PROGRAM MAIN
VAR
	fbSocketConnect   	: FB_SocketConnect;(*TCP/IP建立连接的功能块*)
	fbSocketSend      	: FB_SocketSend;(*TCP/IP的发送功能块*)
	fbSocketReceive   	: FB_SocketReceive;(*TCP/IP的写入的功能块*)
	fbSocketClose     	: FB_SocketClose;(*TCP/IP的关闭建立连接的功能块*)
    bExecute          	: BOOL;(*TCP/IP建立连接的执行位*)
    hSocket           	: T_HSOCKET;(*TCP/IP的句柄*)
	arrSendData			: ARRAY[1..4] OF WORD := [16#1111, 16#2222, 16#3333, 16#4444];(*TCP/IP发送数组*)
	bSend				: BOOL;(*TCP/IP发送的执行位*)
	bRecieve          	: BOOL;(*TCP/IP接收的执行位*)
	arrRecieveData    	: ARRAY[1..4] OF WORD;(*TCP/IP接收数组*)
	bClose            	: BOOL;(*TCP/IP关闭连接的执行位*)
END_VAR

/////////////////////////////////////////////////////////
//注意：/////////////////////////////////////////////////
//该例程序仅供初学者入门学习使用/////////////////////////
//差错在所难免，无法保证绝对正确并完全满足您的使用需求///
//欢迎您提出改进建议。联系邮箱：Support@Beckhoff.com.cn//
/////////////////////////////////////////////////////////

fbSocketConnect(
	sSrvNetId:= , 
	sRemoteHost:='169.254.0.1', //TCP/IP Server的IP地址169.254.0.1
	nRemotePort:=6000 , 		//TCP/IP Server的I端口号6000
	bExecute:= bExecute, 		//TCP/IP连接的执行位*)
	tTimeout:=T#1S , 
	bBusy=> , 
	bError=> , 
	nErrId=> , 
	hSocket=>hSocket );			//通过SocketConnect获取句柄，供后续FB使用
	
fbSocketSend(
	sSrvNetId:= , 
	hSocket:=hSocket , 			//TCP/IP的句柄
	cbLen:=SIZEOF(arrSendData) ,//TCP/IP发送数据的长度
	pSrc:=ADR (arrSendData), 	//TCP/IP发送数据的指针起始地址
	bExecute:=bSend, 			//TCP/IP发送的执行位
	tTimeout:= T#1S, 
	bBusy=> , 
	bError=> , 
	nErrId=> );
	
fbSocketReceive(
	sSrvNetId:= , 
	hSocket:=hSocket , 				//TCP/IP的句柄
	cbLen:=SIZEOF(arrRecieveData) , //TCP/IP接收数据的长度
	pDest:=ADR (arrRecieveData) , 	//TCP/IP接收数据的指针起始地址
	bExecute:=bRecieve, 			//TCP/IP接收的执行位
	tTimeout:= T#1S , 
	bBusy=> , 
	bError=> , 
	nErrId=> , 
	nRecBytes=> );
	
fbSocketClose(
	sSrvNetId:= , 
	hSocket:=hSocket , 			//TCP/IP的句柄
	bExecute:=bClose , 			//TCP/IP关闭连接执行位
	tTimeout:=T#1S , 
	bBusy=> , 
	bError=> , 
	nErrId=> );

END_PROGRAM
